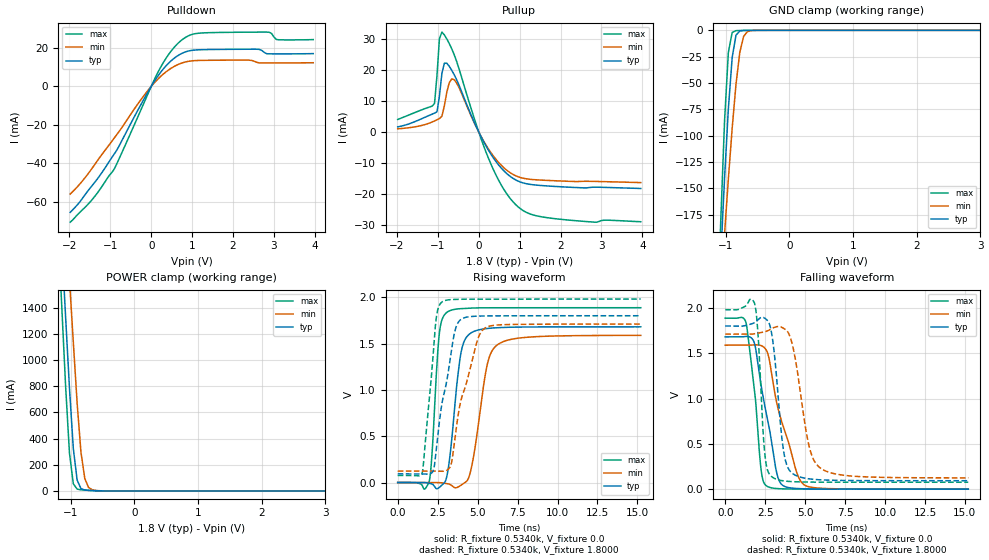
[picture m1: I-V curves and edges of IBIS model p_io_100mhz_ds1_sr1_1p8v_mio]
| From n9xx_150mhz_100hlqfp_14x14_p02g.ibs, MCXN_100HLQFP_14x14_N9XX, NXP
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[Model] p_io_100mhz_ds1_sr1_1p8v_mio
|   Model p_io_100mhz_ds1_sr1_1p8v_mio
| This model was characterised for following simulation conditions:
| External (pad) voltage:
|   - Typ: 1.8V,   - Min: 1.71V,   - Max: 1.98V
| Library cells for typ/min/max conditions are connected as defined below:
|  pad - External Pad
|  ipp_do_lv - Core Input
|  ipp_obe_lv - Output Buffer Enable
|  IOGC - NC
|  REFH3V3 - REFH3V3
|  REFL3V3 - REFL3V3
|  ZI - NC
|  abut_ncal_vddio[1] - vssio vddio vddio
|  abut_ncal_vddio[2] - vddio vddio vssio
|  abut_ncal_vddio[3] - vddio
|  abut_ncal_vddio[4] - vssio vddio vddio
|  abut_ncal_vddio[5] - vddio vddio vssio
|  abut_ncal_vddio[6] - vddio
|  abut_pcal_vddio[1] - vssio
|  abut_pcal_vddio[2] - vddio vssio vddio
|  abut_pcal_vddio[3] - vssio
|  abut_pcal_vddio[4] - vssio
|  abut_pcal_vddio[5] - vddio vssio vddio
|  abut_pcal_vddio[6] - vssio
|  ipp_do_1p8v - ipp_do_1p8v
|  ipp_dse_lv - vdd_lv
|  ipp_eftd_lv - NC
|  ipp_ina_mux_vddio - NC
|  ipp_ina_mux_vddio[0] - NC
|  ipp_ina_mux_vddio[1] - NC
|  ipp_ina_r0_vddio - NC
|  ipp_ina_r0a_vddio - NC
|  ipp_ina_r0b_vddio - NC
|  ipp_ina_r0c_vddio - NC
|  ipp_ina_r0d_vddio - NC
|  ipp_ina_r0e_vddio - NC
|  ipp_ina_r0f_vddio - NC
|  ipp_ina_r300_vddio - NC
|  ipp_ina_r300a_vddio - NC
|  ipp_ina_r300b_vddio - NC
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Model_type I/O
Polarity   Non-Inverting
Enable   Active-High
Vinl =   0.5400V
Vinh =   1.2600V
Vmeas =  0.9000V
Cref =   30.0000pF
Rref =   1.0000M
Vref =   1.8000V
C_comp   1.3623pF   1.2981pF   1.4425pF
|C_comp_pullup   0.7130pF   0.7389pF   0.6867pF
|C_comp_pulldown   0.5818pF   0.6363pF   0.5437pF
[Model Spec]
| variable   typ   min   max
Vinh   1.2600V   1.1970V   1.3860V
Vinl   0.5400V   0.5130V   0.5940V
[Temperature Range]   25.0000   0.1250k   -40.0000
[Voltage Range]   1.8000V   1.7100V   1.9800V
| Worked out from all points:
|   slope of the pulldown table from 0 to 0.27 V, typ, clamps not added: 32.1 ohm
|   slope of the pullup table from 0 to 0.27 V, typ, clamps not added: 40.8 ohm
|   GND clamp passes 1 mA (typ) near -0.79 V on its own axis
|   POWER clamp passes 1 mA (typ) near -0.56 V on its own axis
|   rising waveform, R_fixture 0.5340k, V_fixture 0.0: 20-80 % time 602ps typ, 817ps min, 376ps max; typ from 0 V to 1.68 V
|   rising waveform, R_fixture 0.5340k, V_fixture 1.8000: 20-80 % time 932ps typ, 1.21ns min, 574ps max; typ from 0.093 V to 1.8 V
|   falling waveform, R_fixture 0.5340k, V_fixture 0.0: 20-80 % time 989ps typ, 1.35ns min, 603ps max; typ from 1.68 V to 0 V
|   falling waveform, R_fixture 0.5340k, V_fixture 1.8000: 20-80 % time 546ps typ, 868ps min, 349ps max; typ from 1.8 V to 0.093 V
[Pulldown]
|Voltage   I(typ)   I(min)   I(max)
-1.98V    -65.51mA   -56mA      -70.63mA
-1.44V    -51.49mA   -42.44mA   -58.8mA
-900mV    -35.05mA   -26.74mA   -42.86mA
-240mV    -8.99mA    -6.551mA   -11.63mA
180mV     5.909mA    4.185mA    8.006mA
480mV     13.23mA    9.376mA    18.24mA
780mV     17.5mA     12.4mA     24.7mA
1.2V      19.11mA    13.55mA    27.78mA
2.58V     19.37mA    12.56mA    28.27mA
2.82V     17.04mA    12.25mA    28.29mA
3.06V     16.96mA    12.25mA    24.43mA
3.96V     17.09mA    12.34mA    24.37mA
[Pullup]
|Voltage   I(typ)   I(min)   I(max)
-1.98V    1.636mA    1mA        4.028mA
-1.08V    6.077mA    3.554mA    9.208mA
-1.02V    6.51mA     3.931mA    18.29mA
-960mV    11.61mA    4.325mA    30.19mA
-900mV    18.94mA    5.078mA    32.34mA
-840mV    22.24mA    8.431mA    31.43mA
-720mV    21.27mA    15.96mA    28.62mA
-600mV    18.54mA    16.92mA    25.03mA
240mV     -5.971mA   -5.553mA   -8.582mA
900mV     -15.52mA   -14.17mA   -23.51mA
1.68V     -17.51mA   -15.71mA   -27.79mA
3.96V     -18.32mA   -16.41mA   -29.09mA
[GND_clamp]
|Voltage   I(typ)   I(min)   I(max)
-1.98V    -1.537A    -1.19A     -2.019A
-1.14V    -294.9mA   -305.1mA   -290.2mA
-1.08V    -215.7mA   -248.6mA   -182.3mA
-1.02V    -141mA     -193.8mA   -86.65mA
-960mV    -74.83mA   -141.5mA   -21.03mA
-900mV    -25.88mA   -93.07mA   -2.012mA
-840mV    -4.609mA   -51.31mA   -311uA
-780mV    -637.2uA   -20.91mA   -159.7uA
-720mV    -151.2uA   -5.716mA   -109.9uA
-660mV    -72.83uA   -1.219mA   -73.5uA
-480mV    -11.41uA   -25.38uA   -9.438uA
3.96V     0A         0A         0A
[POWER_clamp]
|Voltage   I(typ)   I(min)   I(max)
-1.98V    9.576A     9.287A     10.07A
-1.2V     2.409A     3.037A     2.006A
-1.14V    1.864A     2.56A      1.395A
-1.08V    1.321A     2.084A     791mA
-1.02V    782.7mA    1.609A     287.5mA
-960mV    325.1mA    1.137A     54.65mA
-900mV    82.58mA    671mA      14.08mA
-840mV    18.02mA    296.8mA    8.778mA
-780mV    6.907mA    95.14mA    6.356mA
-720mV    4.149mA    25.95mA    4.381mA
-660mV    2.634mA    7.923mA    2.736mA
3.96V     0A         0A         0A
[Ramp]
| variable   typ   min   max
dV/dt_r  1.0081/0.6015n   0.9529/0.8166n   1.1320/0.3762n
dV/dt_f  1.0242/0.5458n   0.9513/0.8676n   1.1422/0.3494n
R_load = 0.5340k
[Rising Waveform]
R_fixture= 0.5340k
V_fixture= 0.0
V_fixture_min= 0.0
V_fixture_max= 0.0
|time   V(typ)   V(min)   V(max)
0s        464.8pV    171.6nV    14.01pV
1.962ns   -8.084mV   270.5uV    3.573mV
2.153ns   -16.4mV    568.5uV    322.9mV
2.592ns   -54.81mV   -894.4uV   1.589V
3.095ns   82.89mV    -12.13mV   1.839V
3.912ns   1.352V     -34.89mV   1.877V
4.494ns   1.603V     78.2mV     1.882V
5.58ns    1.662V     1.254V     1.886V
6.159ns   1.67V      1.475V     1.886V
15.21ns   1.68V      1.588V     1.887V
[Rising Waveform]
R_fixture= 0.5340k
V_fixture= 1.8000
V_fixture_min= 1.7100
V_fixture_max= 1.9800
|time   V(typ)   V(min)   V(max)
0s        92.99mV    124mV      76.26mV
1.542ns   93.33mV    124mV      109.4mV
2.258ns   145.5mV    124.2mV    1.475V
2.473ns   452mV      123.3mV    1.84V
2.781ns   865.6mV    121.3mV    1.95V
3.336ns   1.392V     193.2mV    1.974V
3.724ns   1.709V     661.1mV    1.977V
4.93ns    1.795V     1.503V     1.98V
5.396ns   1.797V     1.659V     1.98V
15.21ns   1.8V       1.71V      1.98V
[Falling Waveform]
R_fixture= 0.5340k
V_fixture= 0.0
V_fixture_min= 0.0
V_fixture_max= 0.0
|time   V(typ)   V(min)   V(max)
0s        1.68V      1.589V     1.887V
1.303ns   1.685V     1.588V     1.835V
1.832ns   1.608V     1.592V     1.093V
2.246ns   1.144V     1.584V     212mV
2.571ns   836.3mV    1.533V     37.41mV
3.181ns   212.8mV    987.8mV    7.481mV
3.399ns   85.03mV    826.1mV    4.932mV
4.47ns    7.435mV    186.3mV    992uV
4.954ns   3.9mV      46.3mV     566.7uV
15.21ns   35.51uV    84.29uV    22.09uV
[Falling Waveform]
R_fixture= 0.5340k
V_fixture= 1.8000
V_fixture_min= 1.7100
V_fixture_max= 1.9800
|time   V(typ)   V(min)   V(max)
0s        1.8V       1.71V      1.98V
1.851ns   1.839V     1.715V     2.04V
2.063ns   1.871V     1.721V     1.679V
2.473ns   1.886V     1.736V     395.8mV
2.943ns   1.677V     1.775V     133mV
3.635ns   440.6mV    1.776V     91.77mV
4.21ns    173.3mV    1.588V     82.91mV
5.215ns   114.5mV    499.9mV    78.23mV
5.948ns   103.2mV    233.6mV    77.18mV
15.21ns   93.04mV    124.4mV    76.29mV
